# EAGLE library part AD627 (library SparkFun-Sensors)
Hall-effect-based isolated linear current sensor PROTO: IC-13132
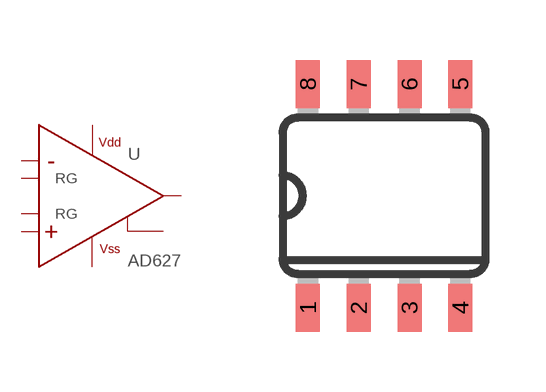
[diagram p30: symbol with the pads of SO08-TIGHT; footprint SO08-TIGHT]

Designator prefix U

## AD627SOIC (PROD_ID: IC-13132; VALUE: AD627)  [SO08-TIGHT]
1  RG
2  IN-
3  IN+
4  VS-
5  REF
6  OUTPUT
7  VS+
8  RG

## Footprint SO08-TIGHT (pad centres in mm)
smd 0.6 x 1.2: 1 -1.905,-2.8; 2 -0.635,-2.8; 3 0.635,-2.8; 4 1.905,-2.8; 5 1.905,2.8; 6 0.635,2.8; 7 -0.635,2.8; 8 -1.905,2.8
